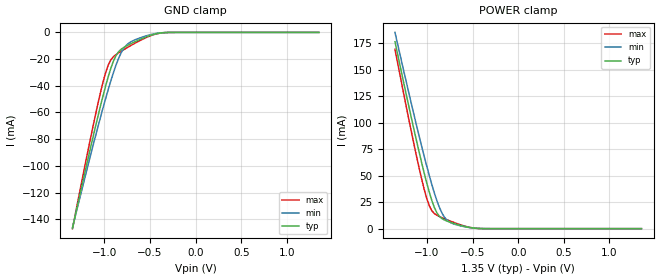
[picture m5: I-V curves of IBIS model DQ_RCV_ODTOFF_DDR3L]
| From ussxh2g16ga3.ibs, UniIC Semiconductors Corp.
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|   Model DQ_RCV_ODTOFF_DDR3L
[Model] DQ_RCV_ODTOFF_DDR3L
Model_type Input
Vinl =  0.540V
Vinh =  0.810V
C_comp   0.966pF   0.965pF   0.967pF
[Model Spec]
Vinh   0.810V   0.776V   0.860V
Vinl   0.540V   0.506V   0.590V
[Temperature Range]   25.000   95.000   -40.000
[Voltage Range]   1.350V   1.283V   1.450V
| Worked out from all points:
|   GND clamp passes 1 mA (typ) near -0.43 V on its own axis
|   POWER clamp passes 1 mA (typ) near -0.52 V on its own axis
[GND_clamp]
|Voltage   I(typ)   I(min)   I(max)
-1.35V    -146.9mA   -146.3mA   -147.1mA
-1.126V   -78.8mA    -85.17mA   -70.77mA
-1.014V   -47.25mA   -56.31mA   -36.92mA
-958mV    -33.17mA   -42.77mA   -24.44mA
-930mV    -26.97mA   -36.36mA   -20.61mA
-874mV    -17.51mA   -24.69mA   -16.72mA
-818mV    -12.71mA   -15.46mA   -14.21mA
-762mV    -10.26mA   -9.751mA   -11.88mA
-706mV    -8.307mA   -6.907mA   -9.644mA
-538mV    -3.274mA   -2.499mA   -3.731mA
-398mV    -591.2uA   -439.3uA   -663.7uA
1.35V     0A         0A         0A
[POWER_clamp]
|Voltage   I(typ)   I(min)   I(max)
-1.35V    176.6mA    185.4mA    169.4mA
-1.198V   115.5mA    128.2mA    103.2mA
-1.114V   83.04mA    97.6mA     68.48mA
-1.058V   62.42mA    77.92mA    46.98mA
-1.002V   43.19mA    59.09mA    28.56mA
-946mV    26.54mA    41.57mA    16.92mA
-890mV    14.85mA    26.22mA    12.66mA
-834mV    9.439mA    14.55mA    10.39mA
-778mV    7.089mA    7.901mA    8.361mA
-638mV    3.198mA    2.764mA    3.815mA
-414mV    126.6uA    165.9uA    94.28uA
1.35V     0A         0A         0A
